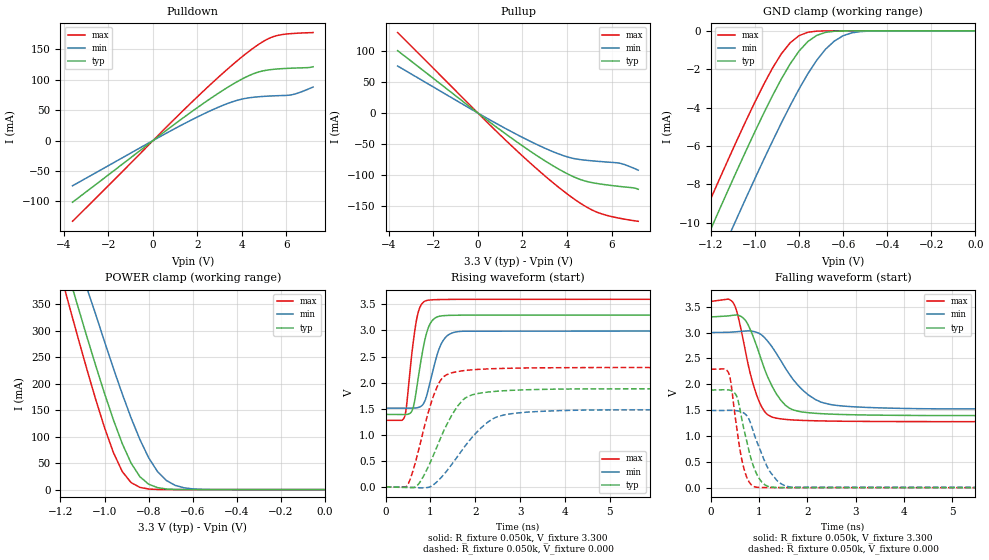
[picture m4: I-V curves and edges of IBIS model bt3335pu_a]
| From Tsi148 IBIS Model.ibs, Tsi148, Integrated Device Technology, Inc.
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|   MODEL bt3335pu_a
[Model]   bt3335pu_a
Model_type   I/O
Vinl  = 0.8V
Vinh  = 2.0V
Vref  = 0.0V
Rref  = 1k
Cref  = 10pF
Vmeas = 1.65V
| Values for delay from A to PAD (Tdo) are determined using
| Vref, Cref, Rref, and Vmeas.
|   INPUT TRANSITION ON DRIVER INPUT = 0.1ns
|   typ   min   max
| Tdo (rise)   1.64n   1.15n   2.33n
| Tdo (fall)   1.50n   1.12n   2.04n
|   INPUT TRANSITION ON DRIVER INPUT = 1.0ns
|   typ   min   max
| Tdo (rise)   1.84n   1.30n   2.59n
| Tdo (fall)   1.60n   1.22n   2.16n
|   typ   min   max
C_comp   1.40pF   1.38pF  1.43pF
[Temperature Range]   50.00   125.00   0.00
[Voltage Range]   3.300   3.000   3.600
|   typ   min   max
|[Supply]   VDD   1.80   1.65   1.95
|[Supply]   VDD330   3.30   3.00   3.60
[Add Submodel]
| Submodel Name   Mode
Up.bt3335pu_a   Non-Driving
Dn.bt3335pu_a   Non-Driving
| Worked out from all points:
|   slope of the pulldown table from 0 to 0.495 V, typ, clamps not added: 35.6 ohm
|   slope of the pullup table from 0 to 0.495 V, typ, clamps not added: 36.5 ohm
|   GND clamp passes 1 mA (typ) near -0.80 V on its own axis
|   POWER clamp passes 1 mA (typ) near -0.71 V on its own axis
|   rising waveform, R_fixture 0.050k, V_fixture 3.300: 20-80 % time 232ps typ, 284ps min, 186ps max; typ from 1.4 V to 3.3 V
|   falling waveform, R_fixture 0.050k, V_fixture 3.300: 20-80 % time 511ps typ, 718ps min, 361ps max; typ from 3.3 V to 1.4 V
|   rising waveform, R_fixture 0.050k, V_fixture 0.000: 20-80 % time 629ps typ, 855ps min, 446ps max; typ from 0.008 V to 1.89 V
|   falling waveform, R_fixture 0.050k, V_fixture 0.000: 20-80 % time 294ps typ, 392ps min, 218ps max; typ from 1.89 V to 0.008 V
[Pullup]   | Note: Vtable = Vcc - Vout
| Voltage   I(typ)   I(min)   I(max)
-3.6V     100.5mA    75.69mA    129.6mA
1.15V     -31.05mA   -23.13mA   -40.45mA
2.69V     -69.57mA   -51.4mA    -91.31mA
3.79V     -93.56mA   -67.99mA   -124.2mA
4.56V     -106.6mA   -74.82mA   -144.3mA
5.33V     -113.4mA   -77.65mA   -159.4mA
5.77V     -115.7mA   -78.91mA   -164.7mA
6.43V     -118.5mA   -81.37mA   -169.9mA
6.98V     -120.5mA   -88.65mA   -173.3mA
7.2V      -122.8mA   -92.05mA   -174.4mA
[Pulldown]   | Note: Vtable = Vout
| Voltage   I(typ)   I(min)   I(max)
-3.6V     -101.4mA   -74.42mA   -132.8mA
250mV     6.651mA    4.841mA    8.721mA
1.79V     48.58mA    34.85mA    64.45mA
3.22V     84.27mA    58.99mA    113.1mA
3.77V     96.43mA    66.01mA    130.6mA
4.21V     105mA      69.69mA    143.7mA
4.87V     114mA      72.41mA    161mA
5.42V     117.2mA    73.55mA    171.1mA
5.75V     118.2mA    74.01mA    174mA
6.3V      119.2mA    75.81mA    176.2mA
7.2V      121.4mA    88.09mA    177.7mA
[POWER_Clamp]   | Note: Vtable = Vcc - Vout
| Voltage   I(typ)   I(min)   I(max)
-3.6V     3.946A     3.816A     4.188A
-1.2V     455.7mA    530.2mA    407.9mA
-1.16V    400.6mA    479.4mA    346.3mA
-1.12V    343.9mA    429.2mA    285.8mA
-1.08V    288.1mA    379.7mA    226.7mA
-1.04V    233.7mA    330.1mA    169.8mA
-1V       181.1mA    278.8mA    116.7mA
-920mV    86.97mA    180.7mA    34.22mA
-840mV    24.39mA    94.6mA     4.235mA
-720mV    1.176mA    17.25mA    44uA
-600mV    19uA       1.348mA    0A
0V        0A         0A         0A
[GND_Clamp]   | Note: Vtable = Vout
| Voltage   I(typ)   I(min)   I(max)
-3.6V     -76.49mA   -78.79mA   -75.06mA
-1.28V    -12.45mA   -14.94mA   -10.87mA
-1.24V    -11.4mA    -13.88mA   -9.809mA
-1.2V     -10.35mA   -12.84mA   -8.759mA
-1.12V    -8.273mA   -10.76mA   -6.689mA
-1.08V    -7.253mA   -9.729mA   -5.675mA
-920mV    -3.381mA   -5.752mA   -1.944mA
-840mV    -1.725mA   -3.901mA   -626uA
-760mV    -561uA     -2.244mA   -74uA
-640mV    -23uA      -536uA     -1uA
-520mV    0A         -38uA      0A
0V        0A         0A         0A
[Ramp]
| variable   typ   min   max
  dV/dt_r   1.13/0.63n   0.89/0.85n   1.37/0.45n
  dV/dt_f   1.14/0.51n   0.89/0.71n   1.39/0.36n
R_load = 0.050k
[Rising Waveform]
R_fixture = 0.050k
V_fixture = 3.300
V_fixture_min = 3.000
V_fixture_max = 3.600
|   time   V(typ)   V(min)   V(max)
0s        1.395V     1.515V     1.282V
420ps     1.392V     1.514V     1.341V
470ps     1.395V     1.514V     1.581V
590ps     1.466V     1.514V     2.594V
700ps     1.936V     1.522V     3.248V
790ps     2.432V     1.551V     3.486V
940ps     3.023V     1.831V     3.579V
1.27ns    3.282V     2.791V     3.593V
1.72ns    3.294V     2.986V     3.596V
19.9ns    3.3V       3V         3.6V
[Falling Waveform]
R_fixture = 0.050k
V_fixture = 3.300
V_fixture_min = 3.000
V_fixture_max = 3.600
|   time   V(typ)   V(min)   V(max)
0s        3.3V       3V         3.6V
460ps     3.332V     3.01V      3.578V
560ps     3.333V     3.017V     3.332V
720ps     3.231V     3.028V     2.635V
870ps     2.942V     3.024V     2.031V
1.05ns    2.467V     2.954V     1.577V
1.45ns    1.696V     2.459V     1.336V
2.17ns    1.443V     1.707V     1.299V
2.97ns    1.415V     1.568V     1.289V
19.9ns    1.395V     1.515V     1.282V
[Rising Waveform]
R_fixture = 0.050k
V_fixture = 0.000
V_fixture_min = 0.000
V_fixture_max = 0.000
|   time   V(typ)   V(min)   V(max)
0s        8mV        7mV        10mV
470ps     -4mV       5mV        22mV
720ps     48mV       -7mV       658mV
990ps     466mV      10mV       1.545V
1.2ns     890mV      153mV      2.011V
1.48ns    1.388V     444mV      2.192V
1.72ns    1.67V      729mV      2.23V
2.41ns    1.833V     1.319V     2.27V
3.41ns    1.872V     1.451V     2.286V
19.9ns    1.891V     1.497V     2.292V
[Falling Waveform]
R_fixture = 0.050k
V_fixture = 0.000
V_fixture_min = 0.000
V_fixture_max = 0.000
|   time   V(typ)   V(min)   V(max)
0s        1.891V     1.497V     2.292V
370ps     1.893V     1.5V       2.221V
420ps     1.881V     1.5V       2.016V
540ps     1.764V     1.493V     1.155V
670ps     1.208V     1.457V     441mV
800ps     690mV      1.312V     113mV
960ps     258mV      885mV      18mV
1.23ns    24mV       313mV      13mV
1.67ns    11mV       21mV       11mV
19.9ns    8mV        7mV        10mV
